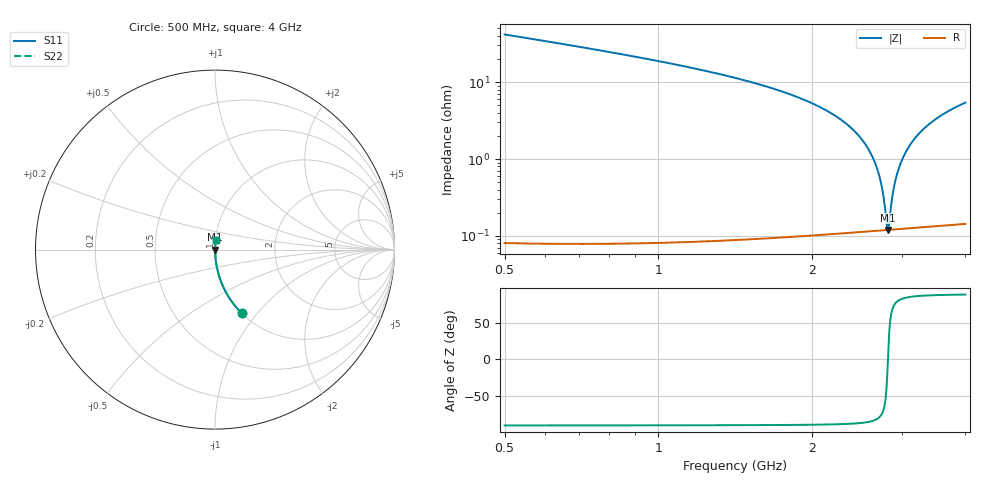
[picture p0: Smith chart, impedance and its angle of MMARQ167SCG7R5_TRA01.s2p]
! MMARQ167SCG7R5_TRA01  S-PARAMETER MODEL  ( General Type )
! Model Generated by TAIYO YUDEN Corporation (http://www.ty-top.com)
! Version 1.0
! TAIYO YUDEN Control No. 160201
! Copyright(c) 2016 TAIYO YUDEN CO.,LTD. All Rights Reserved.
! Product Description (link to TY-COMPAS)
! https://ds.yuden.co.jp/TYCOMPAS/or/detail?pn=MMARQ167SCG7R5CTRA01&u=M
! Products Name : Multilayer Ceramic Capacitors
! Characteristics :
!  Capacitance : 7.5 pF , Rated Voltage : 250V , TCC : CG / C0G
!  Case Size : 1.6 x 0.8 / 0.063 x 0.031 [mm/inch] , Thickness : 0.7 / 0.028 [mm/inch]
!  (Conditions: Temperature = 25 degC , DC Bias Current/Voltage = 0A / 0V)
! External Node Assignments :
!  1  o---| |---o  2
! GND o---------o GND
! Frequency Range : 500MHz  -  4000MHz  [ 401 STEP ]
# MHz S RI R 50
! Freq[MHz].  S11 Real  S11 Imag  S21 Real  S21 Imag  S12 Real  S12 Imag  S22 Real  S22 Imag
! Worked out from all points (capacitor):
!   401 points, 500 MHz to 4 GHz, reference 50 ohm
!   read as one part in series: C = 7.4 pF near 517.5 MHz
!   lowest |Z| = 120 mohm at 2.819 GHz (marker M1)
!   series resonance near 2.82 GHz, so ESL is about 430 pH
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500  0.1483 -0.3545  0.8517 0.3545  0.8517 0.3545  0.1483 -0.3545
736.25  0.0696 -0.253  0.9304 0.253  0.9304 0.253  0.0696 -0.253
1086.25  0.0284 -0.1636  0.9716 0.1636  0.9716 0.1636  0.0284 -0.1636
1672.5  0.0078 -0.0825  0.9922 0.0825  0.9922 0.0825  0.0078 -0.0825
2005  0.0038 -0.0527  0.9962 0.0527  0.9962 0.0527  0.0038 -0.0527
2250  0.00226 -0.0345  0.9977 0.0345  0.9977 0.0345  0.00226 -0.0345
2486.25  0.00149 -0.0192  0.9985 0.0192  0.9985 0.0192  0.00149 -0.0192
2643.75  0.00125 -0.00979  0.9987 0.00979  0.9987 0.00979  0.00125 -0.00979
2696.25  0.00122 -0.0068  0.9988 0.0068  0.9988 0.0068  0.00122 -0.0068
2731.25  0.0012 -0.00485  0.9988 0.00485  0.9988 0.00485  0.0012 -0.00485
2766.25  0.00119 -0.00291  0.9988 0.00291  0.9988 0.00291  0.00119 -0.00291
2801.25  0.00119 -0.00101  0.9988 0.00101  0.9988 0.00101  0.00119 -0.00101
2818.75  0.0012 -6.04e-05  0.9988 6.04e-05  0.9988 6.04e-05  0.0012 -6.04e-05
2836.25  0.0012 0.000879  0.9988 -0.000879  0.9988 -0.000879  0.0012 0.000879
2871.25  0.00121 0.00274  0.9988 -0.00274  0.9988 -0.00274  0.00121 0.00274
2906.25  0.00124 0.00458  0.9988 -0.00458  0.9988 -0.00458  0.00124 0.00458
2950  0.00127 0.00685  0.9987 -0.00685  0.9987 -0.00685  0.00127 0.00685
3011.25  0.00134 0.00997  0.9987 -0.00997  0.9987 -0.00997  0.00134 0.00997
3177.5  0.0016 0.0181  0.9984 -0.0181  0.9984 -0.0181  0.0016 0.0181
3422.5  0.00219 0.0295  0.9978 -0.0295  0.9978 -0.0295  0.00219 0.0295
3685  0.00306 0.041  0.9969 -0.041  0.9969 -0.041  0.00306 0.041
4000  0.00435 0.0539  0.9957 -0.0539  0.9957 -0.0539  0.00435 0.0539
